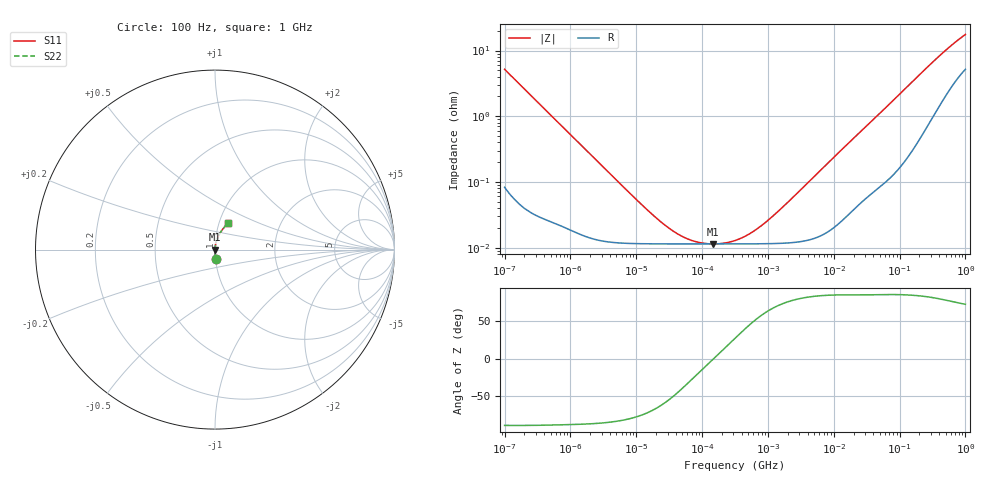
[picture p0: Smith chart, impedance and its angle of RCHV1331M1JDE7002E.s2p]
! RCHV1331M1JDE7002E  S-PARAMETER MODEL  (AEC-Q200 qualified)
! Model Generated by ELNA Corporation (http://www.ty-top.com)
! Version 1.0
! ELNA Control No.240229
! Copyright (c) 2024 ELNA CO.,LTD. All Rights Reserved.
! Products Name : CONDUCTIVE POLYMER HYBRID ALUMINUM ELECTROLYTIC CAPACITORS
! Characteristics :
!  Capacitance  :  330uF  ,  Rated voltage  :  6.3V
!  Operating Temp. Range  :  -55 to +105 degC  ,  Endurance  :  10000hr at 105 degC
!  Dimension D  :  6.3mm  ,  Dimension L  :  7.7mm
! Frequency Range : 100Hz - 1GHz
! External Node Assignments :
!  1  o---| |---o  2
# MHz S RI R 50
!Freq[MHz].  S11 Real  S11 Imag  S21 Real  S21 Imag  S12 Real  S12 Imag  S22 Real  S22 Imag
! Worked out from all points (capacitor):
!   401 points, 100 Hz to 1 GHz, reference 50 ohm
!   read as one part in series: C = 307 uF near 108 Hz
!   lowest |Z| = 11.4 mohm at 147.1 kHz (marker M1)
!   series resonance near 149.2 kHz, so ESL is about 3.7 nH
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0.0001  0.0035 -0.0516  0.9965 0.0516  0.9965 0.0516  0.0035 -0.0516
0.000113  0.0028 -0.0457  0.9972 0.0457  0.9972 0.0457  0.0028 -0.0457
0.000309  0.000586 -0.0168  0.9994 0.0168  0.9994 0.0168  0.000586 -0.0168
0.001488  0.000168 -0.00354  0.9998 0.00354  0.9998 0.00354  0.000168 -0.00354
0.009495  0.000115 -0.000557  0.9999 0.000557  0.9999 0.000557  0.000115 -0.000557
0.022131  0.000114 -0.000235  0.9999 0.000235  0.9999 0.000235  0.000114 -0.000235
0.037368  0.000114 -0.000133  0.9999 0.000133  0.9999 0.000133  0.000114 -0.000133
0.05821  0.000114 -7.73e-05  0.9999 7.73e-05  0.9999 7.73e-05  0.000114 -7.73e-05
0.090678  0.000114 -3.69e-05  0.9999 3.69e-05  0.9999 3.69e-05  0.000114 -3.69e-05
0.147062  0.000114 -1.02e-06  0.9999 1.02e-06  0.9999 1.02e-06  0.000114 -1.02e-06
0.220039  0.000114 2.84e-05  0.9999 -2.84e-05  0.9999 -2.84e-05  0.000114 2.84e-05
0.316228  0.000114 5.86e-05  0.9999 -5.86e-05  0.9999 -5.86e-05  0.000114 5.86e-05
0.512861  0.000114 0.000112  0.9999 -0.000112  0.9999 -0.000112  0.000114 0.000112
0.865964  0.000115 0.0002  0.9999 -0.0002  0.9999 -0.0002  0.000115 0.0002
1.650061  0.000117 0.00039  0.9999 -0.00039  0.9999 -0.00039  0.000117 0.00039
4.704354  0.000136 0.00112  0.9999 -0.00112  0.9999 -0.00112  0.000136 0.00112
69.9842  0.00135 0.0152  0.9987 -0.0152  0.9987 -0.0152  0.00135 0.0152
176.8072  0.005 0.0373  0.995 -0.0373  0.995 -0.0373  0.005 0.0373
395.8221  0.0198 0.0777  0.9802 -0.0777  0.9802 -0.0777  0.0198 0.0777
668.3439  0.0444 0.1156  0.9556 -0.1156  0.9556 -0.1156  0.0444 0.1156
922.5714  0.0666 0.1412  0.9334 -0.1412  0.9334 -0.1412  0.0666 0.1412
1000  0.0728 0.1479  0.9272 -0.1479  0.9272 -0.1479  0.0728 0.1479
